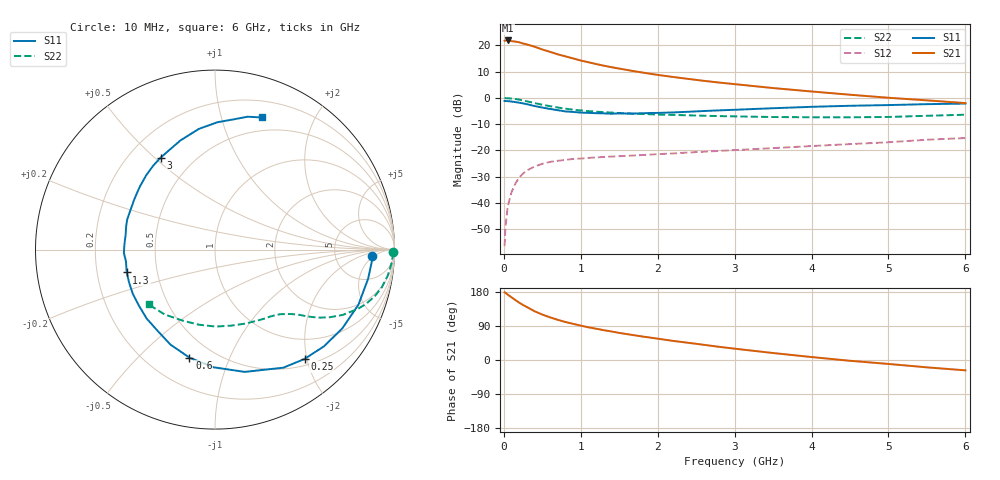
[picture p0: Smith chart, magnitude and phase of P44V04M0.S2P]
! SIEMENS Small Signal Semiconductors
! BFP182
! Si NPN RF Bipolar Junction Transistor in SOT143
! VCE = 4 V  IC = 4 mA
! Common Emitter S-Parameters:  March  1996
# GHz  S  MA  R  50
!  f  S11  S21  S12  S22
! GHz  MAG  ANG  MAG  ANG  MAG  ANG  MAG  ANG
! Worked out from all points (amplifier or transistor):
!   36 points, 10 MHz to 6 GHz, reference 50 ohm
!   highest |S21| = 21.9 dB at 50 MHz (marker M1)
!   |S21| within 3 dB of that: start of sweep to 458 MHz
!   unconditionally stable (mu >= 1): 1.738 GHz to 5.541 GHz
!   at 250 MHz: K = 0.18, MSG = 24.8 dB, |S12| = -28.8 dB
!   at 1.4 GHz: K = 0.86, MSG = 17.0 dB, |S12| = -22.3 dB
!   at 6 GHz: K = 0.96, MSG = 6.7 dB, |S12| = -15.3 dB
!   S11 on the Smith chart (normalised r, x): 10 MHz: 14, -4; 250 MHz: 0.61, -1.96; 600 MHz: 0.37, -0.72; 1.3 GHz: 0.33, -0.11; 3 GHz: 0.33, +0.52; 6 GHz: 0.36, +1.36
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0.01  0.8754 -2.3  12.32 178.6  0.0015 85.9  0.9914 -0.9
0.02  0.8762 -4.4  12.44 177.5  0.0034 84.0  0.9914 -1.7
0.05  0.8685 -10.7  12.47 172.6  0.0085 87.6  0.9872 -4.3
0.15  0.8342 -31.8  11.87 158.1  0.0234 72.8  0.9531 -12.7
0.2  0.8117 -41.6  11.51 151.3  0.0305 68.3  0.927 -16.3
0.25  0.7874 -50.7  10.9 145.2  0.0363 63.5  0.896 -19.6
0.3  0.7603 -59.9  10.47 139.7  0.0416 59.2  0.8638 -22.4
0.4  0.7013 -76.3  9.462 128.6  0.0494 51.9  0.7991 -27.1
0.5  0.6558 -90.7  8.394 119.9  0.0557 46.3  0.7425 -30.5
0.6  0.6184 -103.3  7.567 112.6  0.0605 42.3  0.6978 -32.9
0.7  0.5847 -115.1  6.784 106.1  0.0635 39.2  0.6582 -34.8
0.8  0.5544 -125.1  6.207 100.3  0.066 36.5  0.6261 -36.3
0.9  0.5411 -134.6  5.67 95.4  0.0689 34.8  0.5983 -37.5
1.1  0.5201 -151.6  4.792 86.2  0.0722 31.8  0.5614 -39.8
1.3  0.5082 -165.5  4.118 78.7  0.0753 30.3  0.5365 -41.9
1.6  0.5053 176.2  3.421 68.3  0.079 29.0  0.5088 -45.2
2.2  0.5301 147.9  2.512 50.4  0.0877 28.5  0.4754 -53.5
3  0.5955 120.5  1.835 29.9  0.1015 27.6  0.446 -67.5
3.5  0.6375 107.7  1.544 18.4  0.1108 26.5  0.4333 -77.9
4.5  0.7098 88.9  1.153 -2.1  0.1321 23.1  0.4279 -102.1
5.5  0.7624 76.2  0.9 -19.4  0.1599 19.0  0.4575 -127.8
6  0.7813 70.4  0.799 -27.3  0.1724 15.0  0.4797 -140.4
